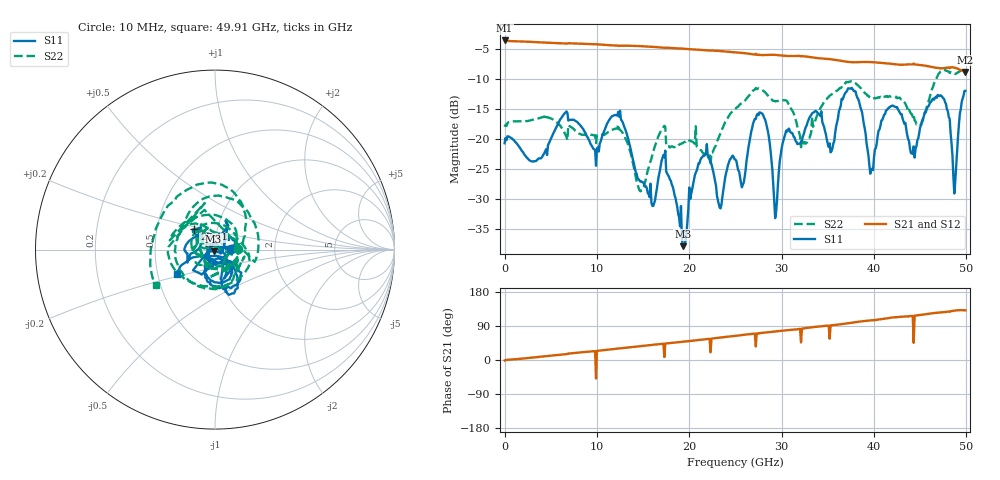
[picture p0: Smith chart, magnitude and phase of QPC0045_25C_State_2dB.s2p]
!File name = QPC0045_25C_State_2dB.s2p
!Date Time: 2024/05/02 05:42:16 AM
!Cal Ref Plane:TRL
!TEMP = 25C
!Vdd(V) = 3.15
!Vss(V) = 0.000
# GHz  S  DB  R  50
!%	Freq(GHz)  S11(dB)  S11(deg)  S21(dB)  S21(deg)  S12(dB)  S12(deg)  S22(dB)  S22(deg)
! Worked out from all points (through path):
!   500 points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, 10 MHz to 49.91 GHz, reference 50 ohm
!   highest |S21| = -3.60 dB at 10 MHz (marker M1); lowest = -8.8 dB at 49.91 GHz (marker M2)
!   lowest |S11| = -37.9 dB at 19.31 GHz (marker M3), VSWR 1.03, Z = 49.2 - j0.963 ohm
!   |S11| at or under -10 dB: start of sweep to end of sweep
!   |S22| runs from -28.8 to -8.3 dB; largest |S21 - S12| = 0.002
!   S11 on the Smith chart (normalised r, x): 10 MHz: 1.20, +0.00; 27.41 GHz: 0.78, +0.18; 49.91 GHz: 0.63, -0.18
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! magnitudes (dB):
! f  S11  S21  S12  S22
! 10 MHz  -20.7  -3.6  -3.6  -18.0
! 8.41 GHz  -18.2  -4.1  -4.1  -19.3
! 12.41 GHz  -16.3  -4.5  -4.5  -18.4
! 14.71 GHz  -27.1  -4.5  -4.5  -28.8
! 16.71 GHz  -26.1  -4.7  -4.7  -19.4
! 19.31 GHz  -37.9  -5.0  -5.0  -20.7
! 21.71 GHz  -22.6  -5.2  -5.2  -22.7
! 23.31 GHz  -31.5  -5.4  -5.4  -19.4
! 25.01 GHz  -23.5  -5.6  -5.6  -15.0
! 25.81 GHz  -27.6  -5.7  -5.7  -13.9
! 27.41 GHz  -15.8  -6.0  -6.0  -11.6
! 29.31 GHz  -33.2  -6.0  -6.0  -13.8
! 30.41 GHz  -19.2  -6.2  -6.2  -13.6
! 33.31 GHz  -15.8  -6.4  -6.4  -16.3
! 35.31 GHz  -22.3  -6.7  -6.7  -12.7
! 37.81 GHz  -12.0  -7.2  -7.2  -10.5
! 39.71 GHz  -25.2  -7.2  -7.2  -13.1
! 41.61 GHz  -14.8  -7.4  -7.4  -12.9
! 44.21 GHz  -22.5  -7.6  -7.6  -16.4
! 47.41 GHz  -13.0  -8.2  -8.2  -8.5
! 48.71 GHz  -29.1  -8.1  -8.1  -9.1
! 49.91 GHz  -12.0  -8.8  -8.8  -8.4
